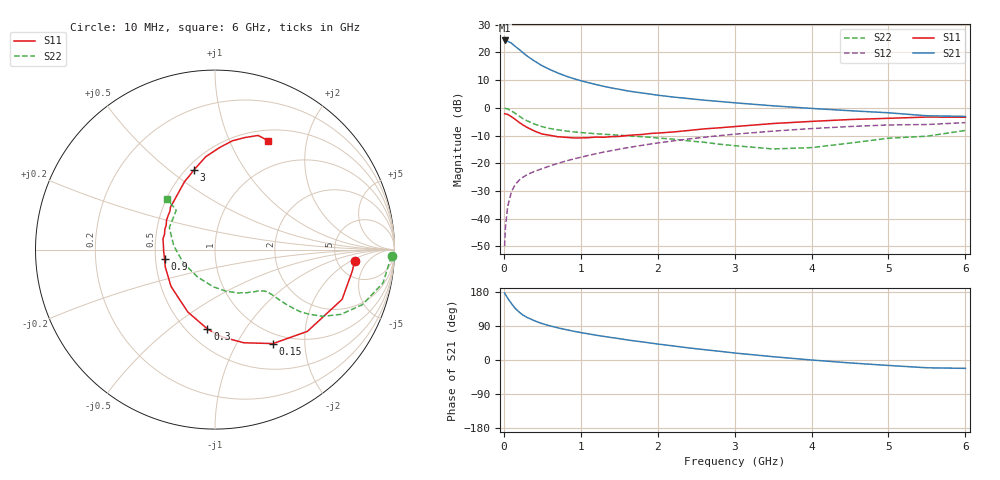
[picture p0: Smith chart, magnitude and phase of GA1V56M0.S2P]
! Infineon Technologies  Discrete & RF Semiconductors
! BF775
! Si NPN RF Bipolar Junction Transistor in SOT23
! VCE = 1.5 V  IC = 6 mA
! Common Emitter S-Parameters:  May  1996
# GHz  S  MA  R  50
!  f  S11  S21  S12  S22
! GHz  MAG  ANG  MAG  ANG  MAG  ANG  MAG  ANG
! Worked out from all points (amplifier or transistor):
!   36 points, 10 MHz to 6 GHz, reference 50 ohm
!   highest |S21| = 24.3 dB at 10 MHz (marker M1)
!   |S21| within 3 dB of that: start of sweep to 188 MHz
!   unconditionally stable (mu >= 1): 678.7 MHz to 4.289 GHz; 5.159 GHz to end of sweep
!   at 250 MHz: K = 0.56, MSG = 22.4 dB, |S12| = -25.0 dB
!   at 1.4 GHz: K = 1.15, MAG = 8.9 dB, |S12| = -15.4 dB
!   at 6 GHz: K = 1.01, MAG = 0.6 dB, |S12| = -5.4 dB
!   S11 on the Smith chart (normalised r, x): 10 MHz: 7.35, -2.36; 150 MHz: 0.85, -1.43; 300 MHz: 0.63, -0.69; 900 MHz: 0.56, -0.07; 3 GHz: 0.55, +0.61; 6 GHz: 0.63, +1.40
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0.01  0.7807 -4.6  16.34 176.7  0.0032 87.8  0.9846 -2.2
0.02  0.7743 -8.9  16.07 173.1  0.0068 86.9  0.9731 -4.5
0.05  0.7604 -21.4  15.83 163.3  0.0168 79.2  0.9545 -11.2
0.1  0.6874 -41.5  14.54 148.5  0.0309 70.5  0.8765 -20.5
0.15  0.6154 -58.3  12.71 135.9  0.0418 63.5  0.7892 -27.2
0.2  0.5434 -72.8  11.23 126.3  0.0496 59.3  0.7074 -31.7
0.25  0.4886 -85.3  9.819 118.5  0.056 56.8  0.6357 -34.5
0.3  0.4445 -95.4  8.609 112.6  0.062 55.8  0.5839 -36.2
0.4  0.3793 -113.5  6.932 103.4  0.0715 54.7  0.5077 -37.5
0.5  0.3355 -128.0  5.702 95.9  0.0801 54.9  0.4546 -38.0
0.6  0.3192 -140.3  4.877 90.1  0.0896 55.8  0.4221 -38.2
0.7  0.3004 -150.9  4.247 85.0  0.0992 56.3  0.4004 -38.4
0.9  0.2863 -169.1  3.375 76.2  0.1188 56.6  0.3688 -39.3
1.1  0.2889 174.5  2.833 69.0  0.1386 56.8  0.3485 -41.4
1.3  0.2938 163.2  2.433 62.3  0.1592 56.2  0.3326 -43.8
1.6  0.3165 148.5  2.024 53.1  0.19 54.4  0.313 -48.8
2.2  0.3659 126.0  1.561 37.1  0.2528 49.2  0.2723 -62.7
3  0.4579 105.0  1.229 18.5  0.3341 39.9  0.2074 -92.7
3.5  0.52 95.7  1.084 8.7  0.3794 33.3  0.1808 -122.6
4.5  0.614 80.9  0.885 -7.7  0.4595 19.9  0.2307 174.8
5.5  0.6799 69.3  0.717 -20.5  0.499 5.7  0.3073 134.6
6  0.6754 64.1  0.699 -22.1  0.5391 1.7  0.3902 133.4
